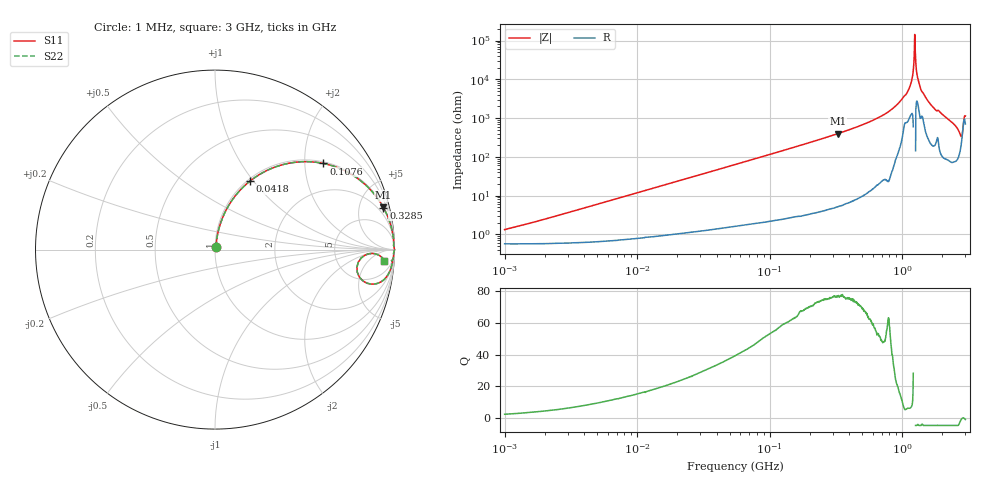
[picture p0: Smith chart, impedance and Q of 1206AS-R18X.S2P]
!s-Parameter Generated by FASTRON Sdn. Bhd.
!FASTRON P/N : 1206AS-R18X
!Keysight Technologies: E4991B_MY54100416_A.01.15
!Date created: Thu Nov 16 09:52:32 2023
!Version  : Rev00 Thu Nov 16 09:52:32 2023
!Data & Calibration Information:
!Freq	S11	S21	S12	S22
!PortZ  Port1:50+j0  Port2:50+j0
!When reading reference impedance value at option line is always used.
! Remarks : This data is being provided solely for informational purposes.
# Hz S dB R 50
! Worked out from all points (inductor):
!   1601 points, 1 MHz to 3 GHz, reference 50 ohm
!   read as one part in series: L = 191 nH near 1.434 MHz
!   highest Q = 77 at 326.9 MHz (marker M1), where L = 193 nH
!   self-resonance near 1.243 GHz
!   S11 on the Smith chart (normalised r, x): 1 MHz: 1.01, +0.02; 41.8 MHz: 1.03, +0.97; 107.6 MHz: 1.05, +2.48; 328.5 MHz: 1.10, +7.99; 3 GHz: 15, -18
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1000000  -37.57 63.9  -0.05 -0.7  -0.05 -0.7  -37.57 63.9
3804036  -26.84 79.7  -0.06 -2.6  -0.06 -2.6  -26.84 79.7
1.447069e7  -15.60 77.4  -0.20 -9.5  -0.20 -9.5  -15.60 77.4
4.180303e7  -7.32 62.8  -1.01 -25.5  -1.01 -25.5  -7.32 62.8
5.477226e7  -5.55 56.7  -1.56 -31.9  -1.56 -31.9  -5.55 56.7
1.076323e8  -2.25 38.5  -4.12 -50.5  -4.12 -50.5  -2.25 38.5
2.083556e8  -0.72 22.2  -8.46 -67.0  -8.46 -67.0  -0.72 22.2
3.268837e8  -0.29 14.1  -12.28 -75.2  -12.28 -75.2  -0.29 14.1
3.285236e8  -0.29 14.0  -12.32 -75.2  -12.32 -75.2  -0.29 14.0
7.925923e8  -0.03 3.9  -23.43 -85.2  -23.43 -85.2  -0.03 3.9
1.097256e9  -0.03 1.2  -33.53 -79.1  -33.53 -79.1  -0.03 1.2
1.159346e9  -0.02 0.8  -37.51 -80.2  -37.51 -80.2  -0.02 0.8
1.212752e9  -0.00 0.3  -44.52 -87.6  -44.52 -87.6  -0.00 0.3
1.249715e9  0.00 -0.0  -61.51 120.1  -61.51 120.1  0.00 -0.0
1.281378e9  -0.01 -0.3  -44.64 81.0  -44.64 81.0  -0.01 -0.3
1.327057e9  -0.02 -0.6  -39.18 77.6  -39.18 77.6  -0.02 -0.6
1.388188e9  -0.03 -1.1  -34.50 77.8  -34.50 77.8  -0.03 -1.1
1.730092e9  -0.06 -3.1  -25.27 80.9  -25.27 80.9  -0.06 -3.1
2.468121e9  -0.22 -8.1  -16.96 75.7  -16.96 75.7  -0.22 -8.1
2.727913e9  -0.91 -12.3  -12.90 58.1  -12.90 58.1  -0.91 -12.3
2.811057e9  -1.91 -9.0  -12.31 31.2  -12.31 31.2  -1.91 -9.0
3e9  -0.48 -3.7  -21.60 48.0  -21.60 48.0  -0.48 -3.7
